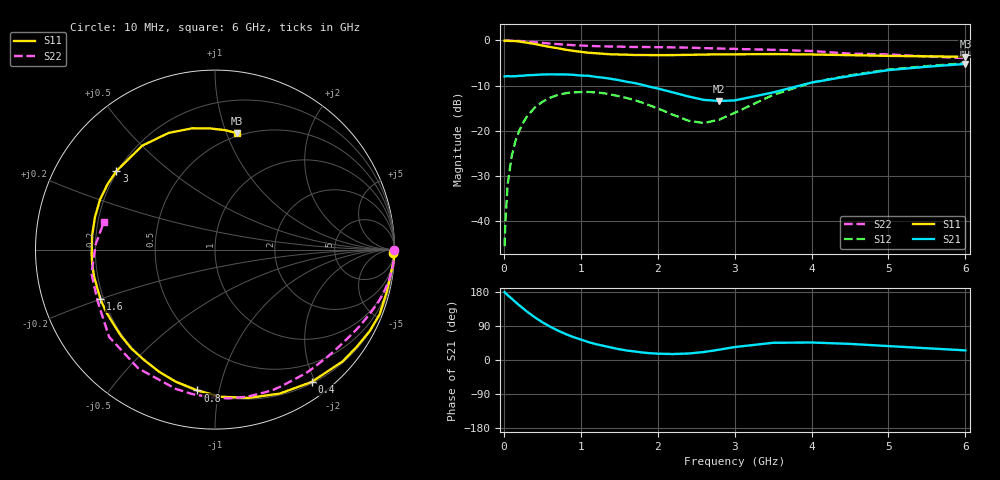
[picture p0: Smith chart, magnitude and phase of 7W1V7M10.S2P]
! Infineon Technologies  Discrete & RF Semiconductors
! BFS17W
! Si NPN RF Bipolar Junction Transistor in SOT323
! VCE = 1.75 V  IC = 0.1 mA
! Common Emitter S-Parameters:  August  1999
# GHz  S  MA  R  50
!  f  S11  S21  S12  S22
! GHz  MAG  ANG  MAG  ANG  MAG  ANG  MAG  ANG
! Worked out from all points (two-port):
!   36 points, 10 MHz to 6 GHz, reference 50 ohm
!   highest |S21| = -5.19 dB at 6 GHz (marker M1); lowest = -13.4 dB at 2.8 GHz (marker M2)
!   |S21| within 3 dB of the highest: start of sweep to 1.27 GHz; 4.384 GHz to end of sweep
!   lowest |S11| = -3.6 dB at 6 GHz (marker M3), VSWR 4.88, Z = 23.6 + j54.3 ohm
!   |S11| at or under -10 dB: nowhere
!   |S22| runs from -3.9 to 0.0 dB; largest |S21 - S12| = 0.4
!   S11 on the Smith chart (normalised r, x): 10 MHz: 26, -88; 400 MHz: 0.22, -1.95; 800 MHz: 0.21, -0.86; 1.6 GHz: 0.19, -0.20; 3 GHz: 0.20, +0.34; 6 GHz: 0.47, +1.09
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0.01  0.9939 -1.2  0.399 179.1  0.0053 84.4  0.9999 0.0
0.02  0.9986 -3.0  0.401 176.5  0.0099 89.9  0.9848 -0.8
0.05  0.9897 -7.1  0.403 171.0  0.0258 85.9  0.9984 -2.3
0.1  0.9855 -13.8  0.401 162.4  0.0515 81.0  0.9963 -4.6
0.2  0.9742 -27.8  0.406 144.5  0.1001 71.3  0.9866 -9.0
0.3  0.9455 -41.2  0.412 128.0  0.1439 62.8  0.9737 -13.2
0.4  0.913 -53.9  0.415 112.9  0.1802 54.3  0.9576 -17.3
0.6  0.8473 -77.2  0.422 88.1  0.2325 40.4  0.925 -24.4
0.8  0.7907 -97.1  0.421 68.8  0.2606 28.7  0.8986 -31.2
1.1  0.7309 -122.7  0.407 47.2  0.2694 15.0  0.8713 -40.7
1.3  0.7108 -137.5  0.387 37.2  0.2608 8.1  0.8596 -47.2
1.6  0.6954 -156.6  0.349 24.9  0.2308 0.4  0.8492 -56.9
2.2  0.6891 173.5  0.266 15.7  0.1506 2.7  0.8389 -77.7
2.6  0.6984 156.5  0.22 21.0  0.122 27.0  0.8227 -92.0
2.8  0.701 148.7  0.214 27.2  0.133 41.6  0.8146 -99.1
3  0.7023 141.4  0.217 34.1  0.1581 52.0  0.8063 -105.6
3.5  0.7068 125.0  0.266 45.4  0.2498 59.1  0.7878 -122.9
4  0.6997 111.7  0.342 46.2  0.3416 54.3  0.7647 -140.5
4.5  0.6876 100.6  0.405 42.5  0.4114 47.1  0.7144 -156.2
5  0.6753 92.1  0.47 36.7  0.4763 40.0  0.7011 -169.1
5.5  0.6677 85.0  0.512 31.0  0.5207 33.2  0.6654 177.5
6  0.6601 79.5  0.55 25.4  0.5604 27.0  0.6381 166.0
